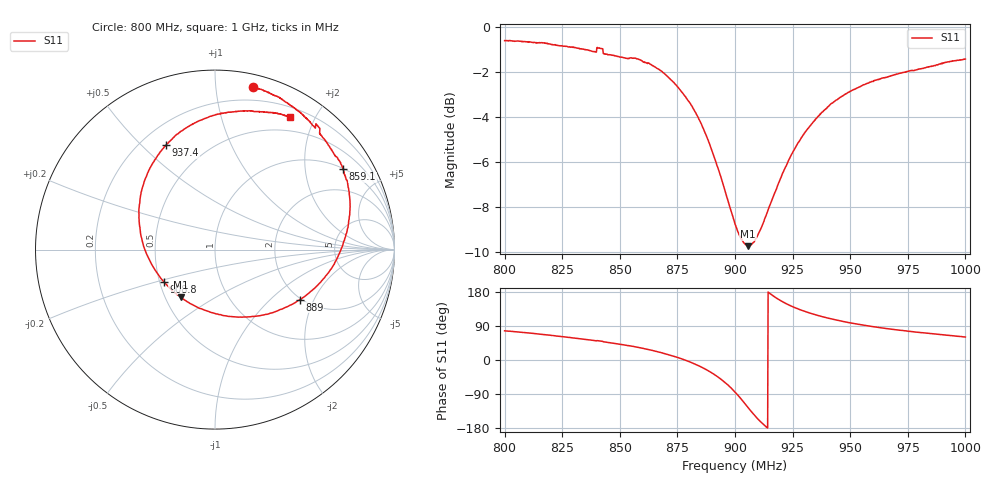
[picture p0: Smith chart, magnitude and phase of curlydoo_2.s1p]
# HZ S RI R 50
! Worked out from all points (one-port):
!   1010 points, 800 MHz to 1 GHz, reference 50 ohm
!   lowest |S11| = -9.7 dB at 905.6 MHz (marker M1), VSWR 1.97, Z = 30.1 - j18 ohm
!   |S11| at or under -10 dB: nowhere
!   S11 on the Smith chart (normalised r, x): 800 MHz: 0.09, +1.25; 859.1 MHz: 1.03, +3.17; 889 MHz: 1.96, -1.57; 908.8 MHz: 0.53, -0.21; 937.4 MHz: 0.30, +0.59; 1 GHz: 0.32, +1.67
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8e8  0.2097 0.9068
8.160555e8  0.3492 0.8525
8.251734e8  0.4309 0.7973
8.388503e8  0.5501 0.6881
8.410307e8  0.5714 0.692
8.438057e8  0.5894 0.6377
8.501486e8  0.6415 0.5662
8.590684e8  0.714 0.447
8.675917e8  0.7516 0.2716
8.751239e8  0.7297 0.0861
8.822596e8  0.6434 -0.1113
8.856293e8  0.5699 -0.2004
8.88999e8  0.4726 -0.2789
8.947472e8  0.26 -0.3658
9.000991e8  0.0326 -0.3626
9.056491e8  -0.1882 -0.2666
9.088206e8  -0.2867 -0.178
9.123885e8  -0.3632 -0.0625
9.161546e8  -0.409 0.0656
9.205153e8  -0.4247 0.204
9.250743e8  -0.4079 0.3337
9.310208e8  -0.3525 0.4719
9.373637e8  -0.2736 0.5821
9.429137e8  -0.1994 0.6515
9.500495e8  -0.1015 0.7115
9.613478e8  0.0449 0.7599
9.750247e8  0.1898 0.7737
9.999999e8  0.4162 0.7382
